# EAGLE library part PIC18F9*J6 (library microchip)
PIC18F97J60 Family 64/80/100-Pin High-Performance, 1-Mbit Flash Microcontrollers with Ethernet Source: http://ww1.microchip.com/downloads/en/DeviceDoc/39762d.pdf
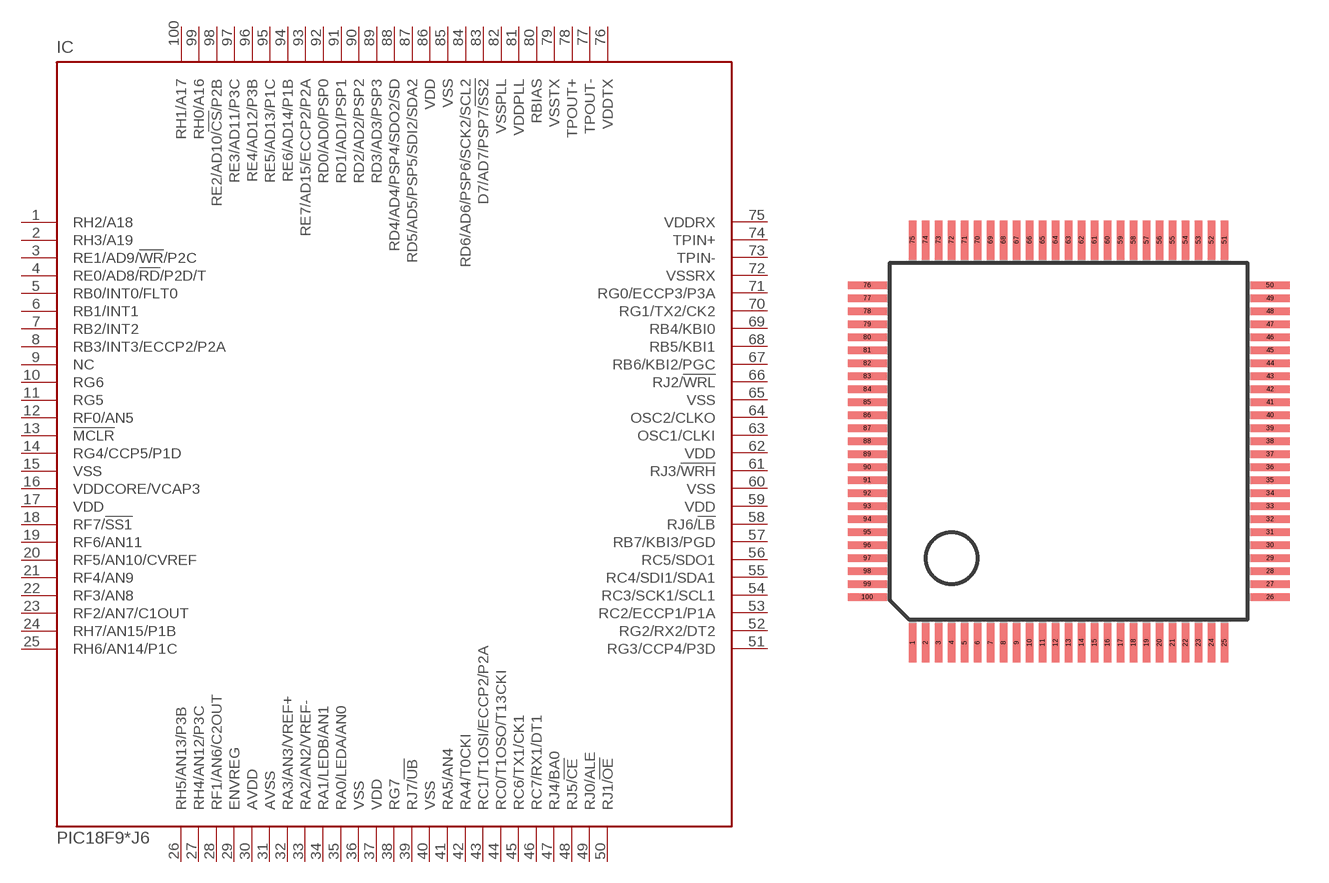
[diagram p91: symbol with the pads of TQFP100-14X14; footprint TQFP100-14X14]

Designator prefix IC

## PIC18F96J60 (MPN: PIC18F96J60-I/PT; OC_FARNELL: 1332292; OC_NEWARK: 56K7316), PIC18F97J60 (MPN: PIC18F97J60-I/PT; OC_FARNELL: 1439573; OC_NEWARK: 56K7318)  [TQFP100-14X14]
1  RH2/A18
2  RH3/A19
3  RE1/AD9/!WR!/P2C
4  RE0/AD8/!RD!/P2D/T
5  RB0/INT0/FLT0
6  RB1/INT1
7  RB2/INT2
8  RB3/INT3/ECCP2/P2A
9  NC  nc
10  RG6
11  RG5
12  RF0/AN5
13  !MCLR  in
14  RG4/CCP5/P1D
15  VSS  pwr
16  VDDCORE/VCAP3
17  VDD  pwr
18  RF7/!SS1
19  RF6/AN11
20  RF5/AN10/CVREF
21  RF4/AN9
22  RF3/AN8
23  RF2/AN7/C1OUT
24  RH7/AN15/P1B
25  RH6/AN14/P1C
26  RH5/AN13/P3B
27  RH4/AN12/P3C
28  RF1/AN6/C2OUT
29  ENVREG  in
30  AVDD  in
31  AVSS  in
32  RA3/AN3/VREF+
33  RA2/AN2/VREF-
34  RA1/LEDB/AN1
35  RA0/LEDA/AN0
36  VSS  pwr
37  VDD  pwr
38  RG7
39  RJ7/!UB
40  VSS
41  RA5/AN4
42  RA4/T0CKI
43  RC1/T1OSI/ECCP2/P2A
44  RC0/T1OSO/T13CKI
45  RC6/TX1/CK1
46  RC7/RX1/DT1
47  RJ4/BA0
48  RJ5/!CE
49  RJ0/ALE
50  RJ1/!OE
51  RG3/CCP4/P3D
52  RG2/RX2/DT2
53  RC2/ECCP1/P1A
54  RC3/SCK1/SCL1
55  RC4/SDI1/SDA1
56  RC5/SDO1
57  RB7/KBI3/PGD
58  RJ6/!LB
59  VDD  pwr
60  VSS  pwr
61  RJ3/!WRH
62  VDD  pwr
63  OSC1/CLKI  in
64  OSC2/CLKO  out
65  VSS  pwr
66  RJ2/!WRL
67  RB6/KBI2/PGC
68  RB5/KBI1
69  RB4/KBI0
70  RG1/TX2/CK2
71  RG0/ECCP3/P3A
72  VSSRX  in
73  TPIN-  in
74  TPIN+  in
75  VDDRX  in
76  VDDTX  in
77  TPOUT-
78  TPOUT+
79  VSSTX  in
80  RBIAS  in
81  VDDPLL  in
82  VSSPLL  in
83  D7/AD7/PSP7/!SS2
84  RD6/AD6/PSP6/SCK2/SCL2
85  VSS  pwr
86  VDD  pwr
87  RD5/AD5/PSP5/SDI2/SDA2
88  RD4/AD4/PSP4/SDO2/SD
89  RD3/AD3/PSP3
90  RD2/AD2/PSP2
91  RD1/AD1/PSP1
92  RD0/AD0/PSP0
93  RE7/AD15/ECCP2/P2A
94  RE6/AD14/P1B
95  RE5/AD13/P1C
96  RE4/AD12/P3B
97  RE3/AD11/P3C
98  RE2/AD10/!CS!/P2B
99  RH0/A16
100  RH1/A17

## PIC18F96J65 (MPN: PIC18F96J65-I/PT; OC_FARNELL: 1564573; OC_NEWARK: 56K7317)  [TQFP100-14X14]
Pads as for TQFP100-14X14

## Footprint TQFP100-14X14 (pad centres in mm)
Thin Quad Flat Pack 14x14 mm
smd 0.27 x 1.5: 1 -6,-7.75; 2 -5.5,-7.75; 3 -5,-7.75; 4 -4.5,-7.75; 5 -4,-7.75; 6 -3.5,-7.75; 7 -3,-7.75; 8 -2.5,-7.75; 9 -2,-7.75; 10 -1.5,-7.75; 11 -1,-7.75; 12 -0.5,-7.75; 13 0,-7.75; 14 0.5,-7.75; 15 1,-7.75; 16 1.5,-7.75; 17 2,-7.75; 18 2.5,-7.75; 19 3,-7.75; 20 3.5,-7.75; 21 4,-7.75; 22 4.5,-7.75; 23 5,-7.75; 24 5.5,-7.75; 25 6,-7.75; 51 6,7.75; 52 5.5,7.75; 53 5,7.75; 54 4.5,7.75; 55 4,7.75; 56 3.5,7.75; 57 3,7.75; 58 2.5,7.75; 59 2,7.75; 60 1.5,7.75; 61 1,7.75; 62 0.5,7.75; 63 0,7.75; 64 -0.5,7.75; 65 -1,7.75; 66 -1.5,7.75; 67 -2,7.75; 68 -2.5,7.75; 69 -3,7.75; 70 -3.5,7.75; 71 -4,7.75; 72 -4.5,7.75; 73 -5,7.75; 74 -5.5,7.75; 75 -6,7.75
smd 1.5 x 0.27: 26 7.75,-6; 27 7.75,-5.5; 28 7.75,-5; 29 7.75,-4.5; 30 7.75,-4; 31 7.75,-3.5; 32 7.75,-3; 33 7.75,-2.5; 34 7.75,-2; 35 7.75,-1.5; 36 7.75,-1; 37 7.75,-0.5; 38 7.75,0; 39 7.75,0.5; 40 7.75,1; 41 7.75,1.5; 42 7.75,2; 43 7.75,2.5; 44 7.75,3; 45 7.75,3.5; 46 7.75,4; 47 7.75,4.5; 48 7.75,5; 49 7.75,5.5; 50 7.75,6; 76 -7.75,6; 77 -7.75,5.5; 78 -7.75,5; 79 -7.75,4.5; 80 -7.75,4; 81 -7.75,3.5; 82 -7.75,3; 83 -7.75,2.5; 84 -7.75,2; 85 -7.75,1.5; 86 -7.75,1; 87 -7.75,0.5; 88 -7.75,0; 89 -7.75,-0.5; 90 -7.75,-1; 91 -7.75,-1.5; 92 -7.75,-2; 93 -7.75,-2.5; 94 -7.75,-3; 95 -7.75,-3.5; 96 -7.75,-4; 97 -7.75,-4.5; 98 -7.75,-5; 99 -7.75,-5.5; 100 -7.75,-6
